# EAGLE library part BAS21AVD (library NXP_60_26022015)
High-voltage switching diodes Triple high-voltage switching diodes, encapsulated in a SOT457 (SC-74) small Surface-Mounted Device (SMD) plastic package. AAL Eindhoven MK
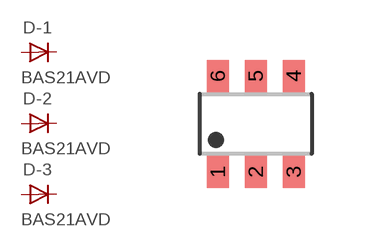
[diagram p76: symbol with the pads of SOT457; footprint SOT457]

Designator prefix D; gates -1=DIODE -2=DIODE -3=DIODE

## BAS21AVD  [SOT457]
1  -1:A  pas
2  -2:A  pas
3  -3:A  pas
4  -3:K  pas
5  -2:K  pas
6  -1:K  pas

## Footprint SOT457 (pad centres in mm)
SOT457 TSOP6: Plastic surface-mounted package; 6 lead JEIDA: SC73 A.K.A. SOT23-6
smd 0.55 x 0.8: 1 -0.95,-1.2; 2 0,-1.2; 3 0.95,-1.2; 4 0.95,1.2; 5 0,1.2; 6 -0.95,1.2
